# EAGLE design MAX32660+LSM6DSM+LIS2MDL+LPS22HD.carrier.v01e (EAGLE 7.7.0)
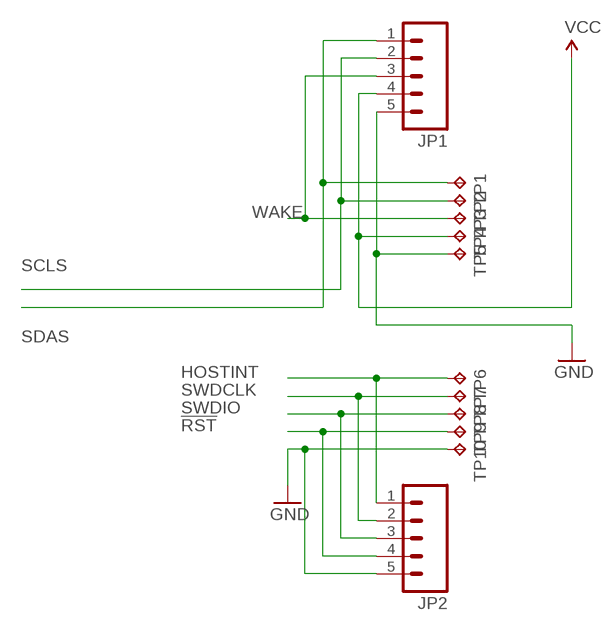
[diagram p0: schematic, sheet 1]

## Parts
JP1  M05NO_SILK  [1X05_NO_SILK]
JP2  M05NO_SILK  [1X05_NO_SILK]
TP1  TPTP08SQ  [TP08SQ]
TP2  TPTP08SQ  [TP08SQ]
TP3  TPTP08SQ  [TP08SQ]
TP4  TPTP08SQ  [TP08SQ]
TP5  TPTP08SQ  [TP08SQ]
TP6  TPTP08SQ  [TP08SQ]
TP7  TPTP08SQ  [TP08SQ]
TP8  TPTP08SQ  [TP08SQ]
TP9  TPTP08SQ  [TP08SQ]
TP10  TPTP08SQ  [TP08SQ]

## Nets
!RST: JP2.4 TP9.TP
GND: JP1.5 JP2.5 TP5.TP TP10.TP
HOSTINT: JP2.1 TP6.TP
SCLS: JP1.2 TP2.TP
SDAS: JP1.1 TP1.TP
SWDCLK: JP2.2 TP7.TP
SWDIO: JP2.3 TP8.TP
VCC: JP1.4 TP4.TP
WAKE: JP1.3 TP3.TP

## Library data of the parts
JP1 JP2 = SparkFun-Connectors:M05: Header 5 Standard 5-pin 0.1" header. Use with straight break away headers (SKU : PRT-00116), right angle break away headers (PRT-00553), swiss pins (PRT-00743), machine pins (PRT-00117), and female headers (PRT-00115). Molex polarized connector foot print use with SKU : PRT-08230 with associated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
TP1-TP10 = testpad:TP: Test pad

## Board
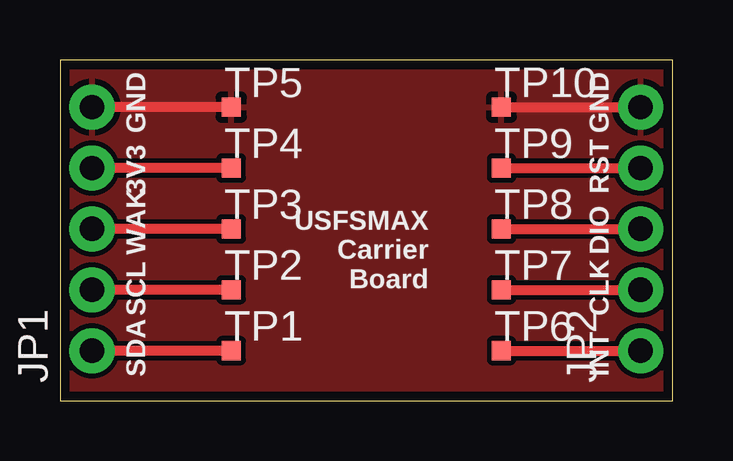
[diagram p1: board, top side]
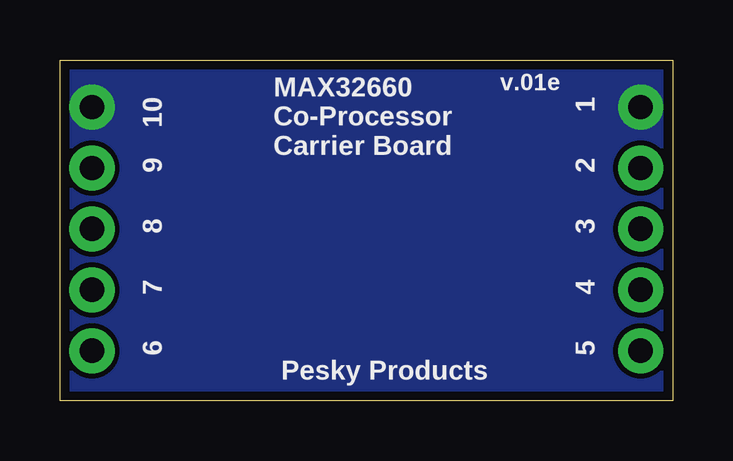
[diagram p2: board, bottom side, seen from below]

Size 25.53 x 14.22 mm. Coordinates in mm from the lower left corner, seen from the top.
Outline: 0,0 25.53,0 25.53,14.22 0,14.22 0,0
Copper layers (1*16): Top 0.035559375mm / dielectric 1.6mm / Bottom 0.035559375mm
Design rules "oshpark-2layer": minimum track width 6mil, minimum drill 10mil, track to track 6mil, track to pad 6mil, pad to pad 6mil, via to via 6mil, smd to smd 6mil, copper to edge 15mil, drill to drill 6mil, minimum pad ring 5mil, minimum via ring 5mil, stop-mask expansion 2.5mil, vias tented up to drill 0mil, thermal gap 10mil

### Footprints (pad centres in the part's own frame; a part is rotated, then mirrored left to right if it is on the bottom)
1X05_NO_SILK = drill 1.016 pad 1.88: 1 0,0; 2 2.54,0; 3 5.08,0; 4 7.62,0; 5 10.16,0
TP08SQ = smd 0.8 x 0.8: TP 0,0

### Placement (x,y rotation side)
JP1  1.33,2.1 90 top
JP2  24.19,2.1 90 top
TP1  7.14,2.1 0 top
TP2  7.14,4.64 0 top
TP3  7.14,7.18 0 top
TP4  7.14,9.72 0 top
TP5  7.14,12.26 0 top
TP6  18.39,2.1 0 top
TP7  18.39,4.64 0 top
TP8  18.39,7.18 0 top
TP9  18.39,9.72 0 top
TP10  18.39,12.26 0 top

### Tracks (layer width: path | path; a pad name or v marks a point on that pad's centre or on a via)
!RST
  Top 0.406: TP9.TP JP2.4
GND
  Top 0.406: TP5.TP JP1.5 | TP10.TP JP2.5
  pour Bottom (isolate 0.203, no thermals): 0,14.22 25.53,14.22 25.53,0 0,0
  pour Top (isolate 0.203): 0,14.22 25.53,14.22 25.53,0 0,0
HOSTINT
  Top 0.406: TP6.TP JP2.1
SCLS
  Top 0.406: TP2.TP JP1.2
SDAS
  Top 0.406: TP1.TP JP1.1
SWDCLK
  Top 0.406: TP7.TP JP2.2
SWDIO
  Top 0.406: TP8.TP JP2.3
VCC
  Top 0.406: TP4.TP JP1.4
WAKE
  Top 0.406: TP3.TP JP1.3

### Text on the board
tPlace: GND | GND | 3V3 | USFSMAX / Carrier / Board | RST | WAK | DIO | SCL | CLK | SDA | INT
bPlace: v.01e | 1 | 10 | 2 | MAX32660 / Co-Processor / Carrier Board | 9 | 3 | 8 | 4 | 7 | 5 | 6 | Pesky Products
